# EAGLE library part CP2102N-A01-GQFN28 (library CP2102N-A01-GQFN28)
SILICON LABS - CP2102N-A01-GQFN28 - USB-UART INTERFACE BRIDGE, QFN-28 Source: Datasheet
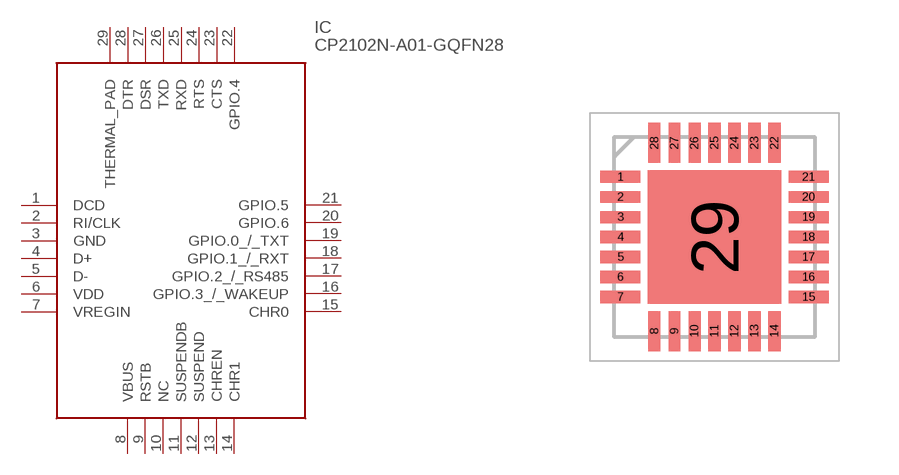
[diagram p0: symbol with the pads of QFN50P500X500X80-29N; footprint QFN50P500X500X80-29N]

Designator prefix IC

## CP2102N-A01-GQFN28 (Arrow_Part_Number: CP2102N-A01-GQFN28; Arrow_Price/Stock: https://www.arrow.com/en/products/cp2102n-a01-gqfn28/silicon-labs; Description: SILICON LABS - CP2102N-A01-GQFN28 - USB-UART INTERFACE BRIDGE, QFN-28; Height: 0.8mm; Manufacturer_Name: Silicon Labs; Manufacturer_Part_Number: CP2102N-A01-GQFN28)  [QFN50P500X500X80-29N]
1  DCD
2  RI/CLK
3  GND
4  D+
5  D-
6  VDD
7  VREGIN
8  VBUS
9  RSTB
10  NC  nc
11  SUSPENDB
12  SUSPEND
13  CHREN
14  CHR1
15  CHR0
16  GPIO.3_/_WAKEUP
17  GPIO.2_/_RS485
18  GPIO.1_/_RXT
19  GPIO.0_/_TXT
20  GPIO.6
21  GPIO.5
22  GPIO.4
23  CTS
24  RTS
25  RXD
26  TXD
27  DSR
28  DTR
29  THERMAL_PAD

## Footprint QFN50P500X500X80-29N (pad centres in mm)
QFN-28_3
smd 1 x 0.3: 1 -2.35,1.5; 2 -2.35,1; 3 -2.35,0.5; 4 -2.35,0; 5 -2.35,-0.5; 6 -2.35,-1; 7 -2.35,-1.5; 15 2.35,-1.5; 16 2.35,-1; 17 2.35,-0.5; 18 2.35,0; 19 2.35,0.5; 20 2.35,1; 21 2.35,1.5
smd 0.3 x 1: 8 -1.5,-2.35; 9 -1,-2.35; 10 -0.5,-2.35; 11 0,-2.35; 12 0.5,-2.35; 13 1,-2.35; 14 1.5,-2.35; 22 1.5,2.35; 23 1,2.35; 24 0.5,2.35; 25 0,2.35; 26 -0.5,2.35; 27 -1,2.35; 28 -1.5,2.35
smd 3.35 x 3.35: 29 0,0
